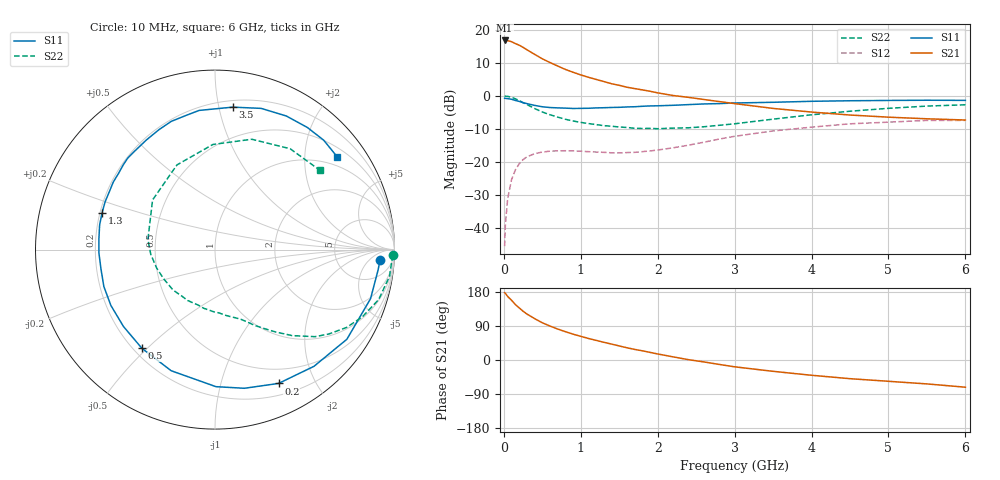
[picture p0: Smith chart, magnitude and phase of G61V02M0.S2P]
! SIEMENS Small Signal Semiconductors
! BFG193
! Si NPN RF Bipolar Junction Transistor in SOT223
! VCE = 1 V  IC = 2 mA
! Common Emitter S-Parameters:  August  1996
# GHz  S  MA  R  50
!  f  S11  S21  S12  S22
! GHz  MAG  ANG  MAG  ANG  MAG  ANG  MAG  ANG
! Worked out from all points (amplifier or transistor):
!   36 points, 10 MHz to 6 GHz, reference 50 ohm
!   highest |S21| = 16.8 dB at 10 MHz (marker M1)
!   |S21| within 3 dB of that: start of sweep to 313 MHz
!   unconditionally stable (mu >= 1): 1.349 GHz to 2.932 GHz; 5.902 GHz to end of sweep
!   at 250 MHz: K = 0.19, MSG = 17.0 dB, |S12| = -19.3 dB
!   at 1.4 GHz: K = 1.04, MAG = 9.2 dB, |S12| = -17.2 dB
!   at 6 GHz: K = 1.00, MAG = -0.3 dB, |S12| = -7.4 dB
!   S11 on the Smith chart (normalised r, x): 10 MHz: 15, -12; 200 MHz: 0.33, -1.53; 500 MHz: 0.23, -0.48; 1.3 GHz: 0.21, +0.15; 3.5 GHz: 0.25, +1.10; 6 GHz: 0.73, +2.79
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0.01  0.9214 -3.6  6.907 177.5  0.0053 88.9  0.9938 -1.8
0.02  0.9156 -7.2  6.886 176.1  0.0111 89.6  0.9872 -3.5
0.05  0.9088 -17.5  6.848 167.6  0.028 80.0  0.9837 -8.7
0.1  0.8885 -34.2  6.623 157.8  0.0538 71.3  0.9534 -17.0
0.15  0.8526 -49.7  6.191 146.2  0.0758 61.7  0.9021 -24.6
0.2  0.8254 -64.6  5.853 137.5  0.0937 54.8  0.8507 -30.7
0.25  0.7899 -78.0  5.434 128.7  0.1084 47.7  0.789 -36.6
0.3  0.7637 -89.6  4.991 121.3  0.1195 42.4  0.7394 -41.0
0.4  0.7177 -109.9  4.261 109.2  0.1333 33.5  0.6439 -48.1
0.5  0.6844 -126.5  3.64 98.2  0.141 26.4  0.5704 -53.6
0.6  0.666 -140.0  3.196 89.6  0.1456 21.8  0.518 -58.1
0.7  0.6583 -151.8  2.832 81.7  0.147 17.9  0.4772 -62.3
0.9  0.6444 -170.3  2.278 68.2  0.1471 12.9  0.4167 -69.2
1.1  0.6496 174.7  1.914 56.8  0.143 10.3  0.3807 -77.7
1.3  0.6617 161.8  1.648 46.7  0.1396 10.1  0.3541 -86.0
1.6  0.6803 146.4  1.352 32.3  0.1387 12.2  0.3325 -101.2
2.2  0.7202 122.2  1.013 8.3  0.1635 19.0  0.3247 -136.1
2.8  0.7643 102.4  0.82 -11.7  0.2218 17.1  0.3586 -175.7
3.5  0.7998 82.9  0.646 -29.9  0.2945 3.5  0.4444 141.5
4.5  0.8438 61.9  0.513 -49.3  0.3778 -18.3  0.5857 91.2
5.5  0.8593 45.2  0.45 -63.1  0.4253 -43.9  0.7008 53.3
6  0.8548 37.3  0.431 -71.8  0.4252 -57.9  0.7328 37.1
